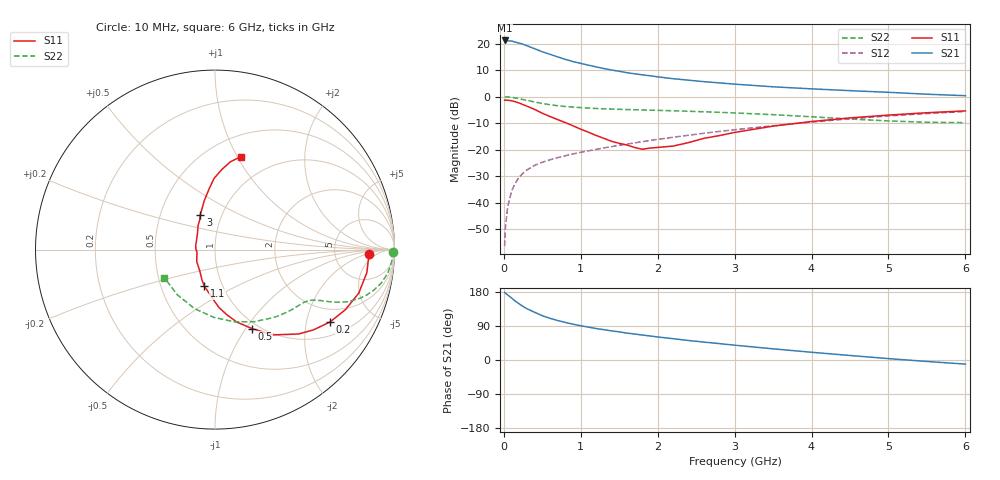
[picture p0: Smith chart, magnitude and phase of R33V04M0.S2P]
! SIEMENS Small Signal Semiconductors
! BFR181
! Si NPN RF Bipolar Junction Transistor in SOT23
! VCE = 3 V  IC = 4 mA
! Common Emitter S-Parameters:  May  1996
# GHz  S  MA  R  50
!  f  S11  S21  S12  S22
! GHz  MAG  ANG  MAG  ANG  MAG  ANG  MAG  ANG
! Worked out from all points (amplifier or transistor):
!   36 points, 10 MHz to 6 GHz, reference 50 ohm
!   highest |S21| = 21.2 dB at 10 MHz (marker M1)
!   |S21| within 3 dB of that: start of sweep to 388.8 MHz
!   unconditionally stable (mu >= 1): 1.218 GHz to 3.046 GHz
!   at 250 MHz: K = 0.37, MSG = 24.3 dB, |S12| = -28.9 dB
!   at 1.4 GHz: K = 1.04, MAG = 13.3 dB, |S12| = -18.9 dB
!   at 6 GHz: K = 0.86, MSG = 3.0 dB, |S12| = -5.6 dB
!   S11 on the Smith chart (normalised r, x): 10 MHz: 13, -3; 200 MHz: 1.46, -2.76; 500 MHz: 0.93, -1.07; 1.1 GHz: 0.82, -0.35; 3 GHz: 0.79, +0.32; 6 GHz: 0.71, +1.04
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0.01  0.8607 -1.8  11.52 178.3  0.0015 84.9  0.9935 -0.8
0.02  0.8568 -3.4  11.37 176.4  0.0033 81.2  0.9853 -1.6
0.05  0.8555 -8.7  11.34 171.7  0.0083 83.9  0.9866 -4.0
0.1  0.8367 -16.9  11.22 163.6  0.0164 80.3  0.9717 -7.8
0.15  0.8004 -24.7  10.7 155.1  0.0234 76.0  0.9455 -11.3
0.2  0.7571 -32.2  10.27 148.1  0.0304 73.3  0.9158 -14.1
0.25  0.7071 -39.3  9.775 141.2  0.036 69.7  0.882 -16.7
0.3  0.6615 -45.3  9.141 135.3  0.0413 67.9  0.8496 -18.7
0.4  0.5746 -55.8  8.038 125.9  0.0503 64.8  0.7933 -21.5
0.5  0.4857 -64.9  7.044 116.8  0.0577 62.7  0.7431 -23.2
0.6  0.4221 -73.2  6.3 110.0  0.0642 61.6  0.7037 -24.4
0.7  0.3688 -79.7  5.636 104.2  0.0706 61.2  0.6738 -25.2
0.8  0.3233 -86.1  5.056 99.1  0.0766 60.9  0.6516 -25.8
0.9  0.2813 -91.5  4.602 94.4  0.083 60.8  0.6354 -26.4
1.1  0.213 -106.0  3.935 86.8  0.0947 61.6  0.6082 -27.6
1.6  0.1222 -146.3  2.84 71.0  0.1274 62.2  0.5708 -31.6
2.2  0.1166 151.3  2.183 56.2  0.1711 61.4  0.5411 -38.6
3  0.2111 112.7  1.724 39.1  0.2372 57.5  0.4925 -50.9
3.5  0.2775 102.6  1.535 29.5  0.2825 53.9  0.4571 -61.5
4.5  0.3972 90.7  1.298 11.9  0.3819 44.0  0.3778 -90.9
5.5  0.4971 80.0  1.112 -3.9  0.4801 31.4  0.3279 -129.6
6  0.5383 74.4  1.042 -10.8  0.5245 24.3  0.3229 -150.9
